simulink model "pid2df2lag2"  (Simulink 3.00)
settings: Solver=ode45  SolverMode=SingleTasking  StartTime=0.0  StopTime=10.0  MaxStep=st_size  RelTol=1e-5  AbsTol=1e-6
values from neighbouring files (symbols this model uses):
  d_through_p = get(MAIN_MENU(19),'Value')    [cback.m]    (also in imcmenu.m = 0)
  Disturb = Setpoint    [mimo_MSF1DF_sim.m]    (also in mimo_MSF2DF_sim.m)
  Satlb = temp1    [cback.m]    (also in imcmenu.m = str2num(satlbs))
  Satub = temp1    [cback.m]    (also in imcmenu.m = str2num(satubs))
  Setpoint = zeros(1,n)    [mimo_MSF1DF_sim.m]    (also in mimo_MSF2DF_sim.m)
undefined symbols (not defined in the file or in its folder): a1, a2, b1, b2, denPd, keps, numPd, pdeadx, Pre_fil_den, Pre_fil_num, XdenPs, XnumPs

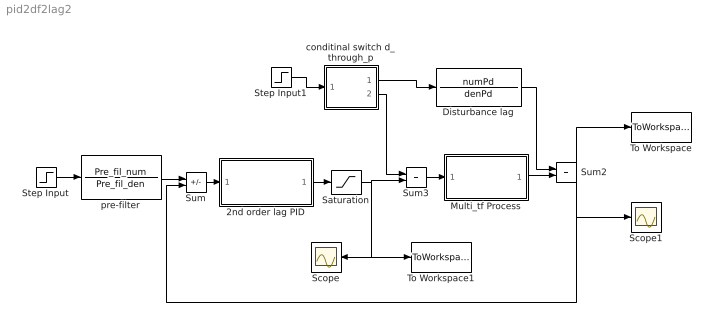
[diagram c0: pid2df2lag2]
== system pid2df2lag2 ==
  2nd order lag PID : Subsystem
  Disturbance lag : TransferFcn  Numerator=numPd  Denominator=denPd
  Multi_tf Process : Subsystem
  Saturation : Saturate  UpperLimit=Satub  LowerLimit=Satlb
  Scope : Scope
  Scope1 : Scope
  Step Input : Step  Time=0  Before=0  After=Setpoint  SampleTime=0
  Step Input1 : Step  Time=0  Before=0  After=Disturb  SampleTime=0
  Sum : Sum  Inputs=+-  SaturateOnIntegerOverflow=on
  Sum2 : Sum  Inputs=++  SaturateOnIntegerOverflow=on
  Sum3 : Sum  Inputs=++  SaturateOnIntegerOverflow=on
  To Workspace : ToWorkspace  VariableName=simout  SampleTime=-1  SaveFormat=Matrix
  To Workspace1 : ToWorkspace  VariableName=effort  SampleTime=-1  SaveFormat=Matrix
  conditinal switch d_through_p : Subsystem  Description=pass input signal through out1 if condition is true.
  pre-filter : TransferFcn  Numerator=Pre_fil_num  Denominator=Pre_fil_den
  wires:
  Step Input/1 -> pre-filter/1
  Sum/1 -> 2nd order lag PID/1(In1)
  pre-filter/1 -> Sum/1
  Disturbance lag/1 -> Sum2/1
  Multi_tf Process/1(Out1) -> Sum2/2
  2nd order lag PID/1(Out1) -> Saturation/1
  Sum3/1 -> Multi_tf Process/1(In1)
  Step Input1/1 -> conditinal switch d_through_p/1(In)
  conditinal switch d_through_p/1(Out2) -> Disturbance lag/1
  conditinal switch d_through_p/2(Out1) -> Sum3/1
  Saturation/1 -> Sum3/2, To Workspace1/1, Scope/1
  Sum2/1 -> Sum/2, To Workspace/1, Scope1/1

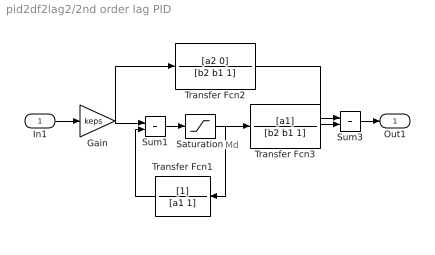
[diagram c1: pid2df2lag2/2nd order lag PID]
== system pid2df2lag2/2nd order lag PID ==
  note: Md
  In1 : Inport  Port=1  PortWidth=-1  SampleTime=-1  DataType=auto
  Gain : Gain  Gain=keps  SaturateOnIntegerOverflow=on
  Saturation : Saturate  UpperLimit=Satub  LowerLimit=Satlb
  Sum1 : Sum  Inputs=++  SaturateOnIntegerOverflow=on
  Sum3 : Sum  Inputs=++  SaturateOnIntegerOverflow=on
  Transfer Fcn1 : TransferFcn  Orientation=left  Numerator=[1]  Denominator=[a1 1]
  Transfer Fcn2 : TransferFcn  Numerator=[a2 0]  Denominator=[b2 b1 1]
  Transfer Fcn3 : TransferFcn  Numerator=[a1]  Denominator=[b2 b1 1]
  Out1 : Outport  Port=1  InitialOutput=0
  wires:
  Gain/1 -> Transfer Fcn2/1, Sum1/1
  Transfer Fcn1/1 -> Sum1/2
  Saturation/1 -> Transfer Fcn1/1, Transfer Fcn3/1
  Sum1/1 -> Saturation/1
  Transfer Fcn3/1 -> Sum3/2
  In1/1 -> Gain/1
  Sum3/1 -> Out1/1
  Transfer Fcn2/1 -> Sum3/1

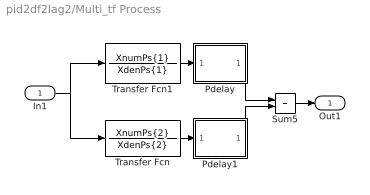
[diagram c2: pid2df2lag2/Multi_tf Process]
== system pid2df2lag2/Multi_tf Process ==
  In1 : Inport  Port=1  PortWidth=-1  SampleTime=-1  DataType=auto
  Pdelay : Subsystem
  Pdelay1 : Subsystem
  Sum5 : Sum  Inputs=++  SaturateOnIntegerOverflow=on
  Transfer Fcn : TransferFcn  Numerator=XnumPs{2}  Denominator=XdenPs{2}
  Transfer Fcn1 : TransferFcn  Numerator=XnumPs{1}  Denominator=XdenPs{1}
  Out1 : Outport  Port=1  InitialOutput=0
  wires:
  Transfer Fcn1/1 -> Pdelay/1(In1)
  Transfer Fcn/1 -> Pdelay1/1(In1)
  In1/1 -> Transfer Fcn1/1, Transfer Fcn/1
  Sum5/1 -> Out1/1
  Pdelay/1(Out1) -> Sum5/1
  Pdelay1/1(Out1) -> Sum5/2

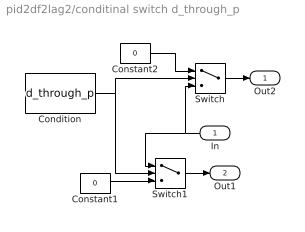
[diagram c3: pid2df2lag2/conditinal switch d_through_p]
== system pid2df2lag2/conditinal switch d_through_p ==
  In : Inport  Orientation=left  Port=1  PortWidth=-1  SampleTime=-1  DataType=auto
  Condition : Constant  Value=d_through_p
  Constant1 : Constant  Value=0
  Constant2 : Constant  Value=0
  Switch : Switch  Threshold=1
  Switch1 : Switch  Threshold=1
  Out2 : Outport  Port=1  InitialOutput=0
  Out1 : Outport  Port=2  InitialOutput=0
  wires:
  In/1 -> Switch/3, Switch1/1
  Condition/1 -> Switch1/2, Switch/2
  Constant1/1 -> Switch1/3
  Constant2/1 -> Switch/1
  Switch/1 -> Out2/1
  Switch1/1 -> Out1/1

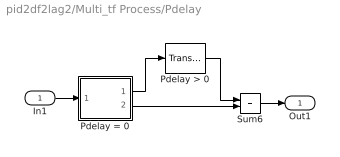
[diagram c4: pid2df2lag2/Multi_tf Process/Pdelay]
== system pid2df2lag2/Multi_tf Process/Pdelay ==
  In1 : Inport  Port=1  PortWidth=-1  SampleTime=-1  DataType=auto
  Pdelay > 0 : TransportDelay  DelayTime=pdeadx(1)  InitialInput=0  BufferSize=1024
  Pdelay = 0 : Subsystem  Description=pass input signal through out1 if condition is true.
  Sum6 : Sum  Inputs=++  SaturateOnIntegerOverflow=on
  Out1 : Outport  Port=1
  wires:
  Pdelay = 0/1(Out2) -> Pdelay > 0/1
  Pdelay > 0/1 -> Sum6/1
  Pdelay = 0/2(Out1) -> Sum6/2
  In1/1 -> Pdelay = 0/1(In)
  Sum6/1 -> Out1/1

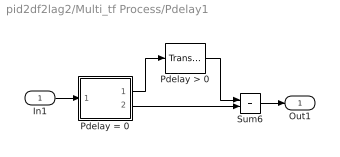
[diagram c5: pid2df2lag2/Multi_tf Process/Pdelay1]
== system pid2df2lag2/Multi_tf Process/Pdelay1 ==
  In1 : Inport  Port=1  PortWidth=-1  SampleTime=-1  DataType=auto
  Pdelay > 0 : TransportDelay  DelayTime=pdeadx(2)  InitialInput=0  BufferSize=1024
  Pdelay = 0 : Subsystem  Description=pass input signal through out1 if condition is true.
  Sum6 : Sum  Inputs=++  SaturateOnIntegerOverflow=on
  Out1 : Outport  Port=1
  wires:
  Pdelay = 0/1(Out2) -> Pdelay > 0/1
  Pdelay > 0/1 -> Sum6/1
  Pdelay = 0/2(Out1) -> Sum6/2
  In1/1 -> Pdelay = 0/1(In)
  Sum6/1 -> Out1/1

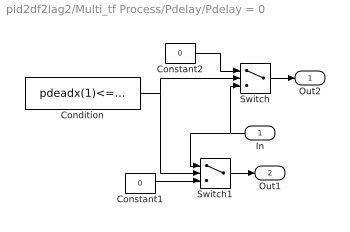
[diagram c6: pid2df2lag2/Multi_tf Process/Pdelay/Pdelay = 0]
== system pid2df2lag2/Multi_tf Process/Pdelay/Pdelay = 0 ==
  In : Inport  Orientation=left  Port=1  PortWidth=-1  SampleTime=-1  DataType=auto
  Condition : Constant  Value=pdeadx(1)<=3*eps
  Constant1 : Constant  Value=0
  Constant2 : Constant  Value=0
  Switch : Switch  Threshold=1
  Switch1 : Switch  Threshold=1
  Out2 : Outport  Port=1  InitialOutput=0
  Out1 : Outport  Port=2  InitialOutput=0
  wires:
  In/1 -> Switch/3, Switch1/1
  Condition/1 -> Switch1/2, Switch/2
  Constant1/1 -> Switch1/3
  Constant2/1 -> Switch/1
  Switch/1 -> Out2/1
  Switch1/1 -> Out1/1

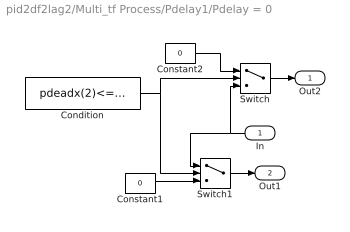
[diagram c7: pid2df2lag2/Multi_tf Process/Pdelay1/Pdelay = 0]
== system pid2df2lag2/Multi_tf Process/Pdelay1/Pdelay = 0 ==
  In : Inport  Orientation=left  Port=1  PortWidth=-1  SampleTime=-1  DataType=auto
  Condition : Constant  Value=pdeadx(2)<=3*eps
  Constant1 : Constant  Value=0
  Constant2 : Constant  Value=0
  Switch : Switch  Threshold=1
  Switch1 : Switch  Threshold=1
  Out2 : Outport  Port=1  InitialOutput=0
  Out1 : Outport  Port=2  InitialOutput=0
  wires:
  In/1 -> Switch/3, Switch1/1
  Condition/1 -> Switch1/2, Switch/2
  Constant1/1 -> Switch1/3
  Constant2/1 -> Switch/1
  Switch/1 -> Out2/1
  Switch1/1 -> Out1/1
